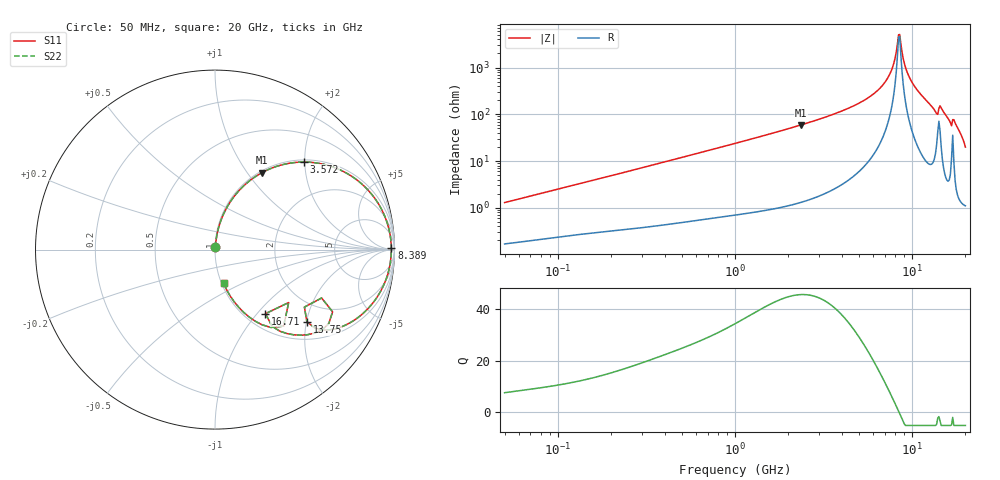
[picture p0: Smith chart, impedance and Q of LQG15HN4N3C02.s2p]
!Murata Part Number: LQG15HN4N3C02
!These Parameters are Measured in Series Mode Connection
!  o--[Z]--o
!Port1  Port2
!  o-------o
!Freq. Start=50[MHz] Stop=20[GHz], 401[Steps]
# Hz S RI R 50
!Freq.(Hz) S11(Real) S11(Imag) S21(Real) S21(Imag) S12(Real) S12(Imag) S22(Real) S22(Imag)
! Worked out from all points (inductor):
!   401 points, 50 MHz to 20 GHz, reference 50 ohm
!   read as one part in series: L = 4.03 nH near 51.52 MHz
!   highest Q = 45.4 at 2.349 GHz (marker M1), where L = 3.98 nH
!   self-resonance near 8.389 GHz
!   S11 on the Smith chart (normalised r, x): 50 MHz: 1.00, +0.03; 3.572 GHz: 1.05, +1.98; 8.389 GHz: open; 13.75 GHz: 1.44, -2.01; 16.71 GHz: 1.23, -1.11; 20 GHz: 1.02, -0.40
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5e7  0.00184 0.0127  0.9982 -0.0127  0.9982 -0.0127  0.00184 0.0127
1.364002e8  0.00382 0.0332  0.9962 -0.0332  0.9962 -0.0332  0.00382 0.0332
3.721004e8  0.0119 0.0875  0.9881 -0.0875  0.9881 -0.0875  0.0119 0.0875
1e9  0.0593 0.2219  0.9407 -0.2219  0.9407 -0.2219  0.0593 0.2219
2.348516e9  0.2615 0.4286  0.7385 -0.4286  0.7385 -0.4286  0.2615 0.4286
2.728004e9  0.333 0.4603  0.667 -0.4603  0.667 -0.4603  0.333 0.4603
3.572216e9  0.4961 0.4879  0.5039 -0.4879  0.5039 -0.4879  0.4961 0.4879
5.769027e9  0.8387 0.3461  0.1613 -0.3461  0.1613 -0.3461  0.8387 0.3461
6.701223e9  0.9234 0.2332  0.0766 -0.2332  0.0766 -0.2332  0.9234 0.2332
7.442007e9  0.9635 0.1354  0.0365 -0.1354  0.0365 -0.1354  0.9635 0.1354
7.901521e9  0.977 0.0737  0.023 -0.0737  0.023 -0.0737  0.977 0.0737
8.389408e9  0.9825 0.00866  0.0175 -0.00866  0.0175 -0.00866  0.9825 0.00866
8.644534e9  0.9819 -0.0248  0.0181 0.0248  0.0181 0.0248  0.9819 -0.0248
9.316812e9  0.9696 -0.1104  0.0304 0.1104  0.0304 0.1104  0.9696 -0.1104
1.004137e10  0.9405 -0.1966  0.0595 0.1966  0.0595 0.1966  0.9405 -0.1966
1.276073e10  0.6972 -0.4331  0.3028 0.4331  0.3028 0.4331  0.6972 -0.4331
1.375312e10  0.5118 -0.4028  0.4882 0.4028  0.4882 0.4028  0.5118 -0.4028
1.460232e10  0.6336 -0.4135  0.3664 0.4135  0.3664 0.4135  0.6336 -0.4135
1.550395e10  0.4774 -0.4769  0.5226 0.4769  0.5226 0.4769  0.4774 -0.4769
1.670968e10  0.2812 -0.3569  0.7188 0.3569  0.7188 0.3569  0.2812 -0.3569
1.774144e10  0.2623 -0.4189  0.7377 0.4189  0.7377 0.4189  0.2623 -0.4189
2e10  0.0475 -0.1868  0.9525 0.1868  0.9525 0.1868  0.0475 -0.1868
